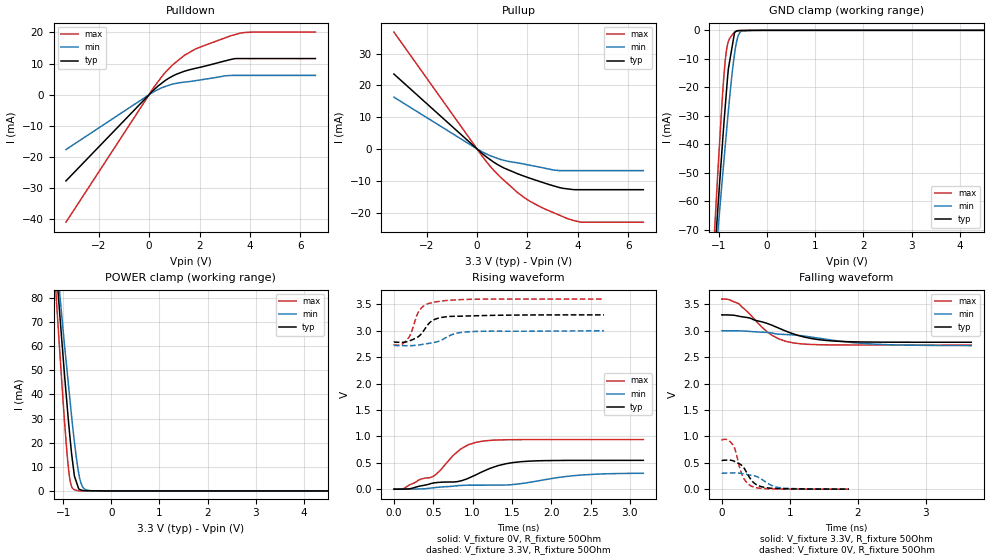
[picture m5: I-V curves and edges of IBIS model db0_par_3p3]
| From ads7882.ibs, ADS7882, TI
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|   db0_par_3p3 Model
[Model]   db0_par_3p3
Model_type   3-state
Polarity   Non-Inverting
Enable   Active-Low
Vmeas = 1.65
Vref = 1.65
Cref = 20pF
Rref = 50
|   typ   min   max
|   (nom PVT)   (Fast PVT)   (slow PVT)
|C_comp from frequency sweep method (F=1.5MHz)
|Average
C_comp   1.719e-12   1.545e-12   1.914e-12
|ON state : BUFFER OUTPUT TURNED HIGH
|C_comp   1.674e-12   1.503e-12   1.875e-12
|OFF state: BUFFER IN HIGH IMPEDANCE
|C_comp   1.764e-12   1.588e-12   1.953e-12
|C_comp from LC tank measurement(L=1nH)
|Resonant Frequency(Hz)   4.480e+09   4.600e+09   4.370e+09
|C_comp   1.263e-12   1.198e-12   1.328e-12
|ON state : BUFFER OUTPUT TURNED HIGH
|Resonant Frequency(Hz)   4.480e+09   4.600e+09   4.370e+09
|C_comp   1.263e-12   1.198e-12   1.328e-12
|OFF state: BUFFER IN HIGH IMPEDANCE
|Resonant Frequency   4.490e+09   4.600e+09   4.090e+09
|C_comp   1.258e-12   1.198e-12   1.516e-12
| Where nom  PVT is Nominal Process,  3.3V,  25C
|   Fast PVT is Strong Process,   3.6V,  -40C
|   Slow PVT is Weak Process,   3V,  85C
[Voltage Range]   3.3   3   3.6
|Ambient Temperature   25   85   -40
|Junction Temperature
[Temperature Range]   25   85   -40
[Pullup Reference]   3.3   3   3.6
[Pulldown Reference]   0   0   0
[Power Clamp Reference]   3.3   3   3.6
[GND Clamp Reference]   0   0   0
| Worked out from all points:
|   slope of the pulldown table from 0 to 0.495 V, typ, clamps not added: 135 ohm
|   slope of the pullup table from 0 to 0.495 V, typ, clamps not added: 154 ohm
|   GND clamp passes 1 mA (typ) near -0.68 V on its own axis
|   POWER clamp passes 1 mA (typ) near -0.68 V on its own axis
|   falling waveform, V_fixture 3.3V, R_fixture 50Ohm: 20-80 % time 703ps typ, 1.15ns min, 433ps max; typ from 3.3 V to 2.78 V
|   rising waveform, V_fixture 0V, R_fixture 50Ohm: 20-80 % time 826ps typ, 1.42ns min, 500ps max; typ from 0 V to 0.545 V
|   rising waveform, V_fixture 3.3V, R_fixture 50Ohm: 20-80 % time 185ps typ, 269ps min, 144ps max; typ from 2.78 V to 3.3 V
|   falling waveform, V_fixture 0V, R_fixture 50Ohm: 20-80 % time 178ps typ, 248ps min, 136ps max; typ from 0.546 V to 0 V
[Pulldown]
|   Voltage   I(typ)   I(min)   I(max)
-3.3V     -27.69mA   -17.63mA   -40.95mA
202.8mV   1.678mA    1.002mA    2.555mA
638.4mV   4.547mA    2.612mA    7.116mA
915.6mV   5.909mA    3.376mA    9.441mA
1.376V    7.461mA    4.003mA    12.49mA
1.916V    8.596mA    4.59mA     14.93mA
3.018V    10.85mA    6.05mA     18.25mA
3.432V    11.59mA    6.179mA    19.34mA
3.644V    11.59mA    6.179mA    19.82mA
4.127V    11.59mA    6.179mA    20.1mA
6.6V      11.59mA    6.179mA    20.1mA
[GND Clamp]
|   Voltage   I(typ)   I(min)   I(max)
-3.3V     -634.8mA   -537.3mA   -767.7mA
-1.136V   -90.43mA   -93.43mA   -83.87mA
-1.056V   -70.52mA   -77.1mA    -59.57mA
-1.01V    -59.08mA   -67.92mA   -45.7mA
-927.6mV  -39.68mA   -51.59mA   -22.91mA
-870mV    -26.75mA   -40.54mA   -10.58mA
-805.2mV  -13.53mA   -28.33mA   -3.894mA
-676.5mV  -750.2uA   -8.253mA   -729.3uA
-650.1mV  -330.5uA   -5.341mA   -460.8uA
-564mV    -97.6uA    -698.5uA   -56.58uA
-360mV    -55.08uA   -511.3nA   0A
6.6V      0A         0A         0A
[Pullup]
|   Voltage   I(typ)   I(min)   I(max)
-3.3V     23.55mA    16.29mA    36.76mA
202.8mV   -1.439mA   -906.1uA   -2.279mA
494.4mV   -3.213mA   -2.04mA    -5.205mA
915.6mV   -5.371mA   -3.274mA   -8.802mA
1.614V    -7.827mA   -4.388mA   -13.76mA
2.053V    -9.089mA   -5.062mA   -16.25mA
2.467V    -10.19mA   -5.705mA   -18.04mA
3.156V    -11.89mA   -6.741mA   -20.46mA
3.846V    -12.81mA   -6.823mA   -22.56mA
4.134V    -12.82mA   -6.823mA   -23.05mA
6.6V      -12.82mA   -6.823mA   -23.05mA
[POWER Clamp]
|   Voltage   I(typ)   I(min)   I(max)
-3.3V     660.3mA    569.4mA    775.2mA
-1.144V   92.02mA    97.34mA    80.17mA
-1.136V   90.18mA    95.79mA    77.92mA
-1.021V   60.73mA    71.04mA    42.87mA
-902.4mV  31.83mA    46.54mA    11.81mA
-852mV    20.98mA    36.39mA    3.781mA
-769.2mV  6.651mA    20.83mA    511.3uA
-696mV    2.004mA    9.587mA    107.3uA
-633mV    404.3uA    3.408mA    6.706uA
-567mV    133.2uA    945.8uA    0A
-429mV    94.19uA    74.67uA    0A
6.6V      0A         0A         0A
[Ramp]
R_load = 50
|   typ   min   max
dV/dt_r   0.327733/8.2648e-10   0.182281/1.43669e-09   0.563152/4.9974e-10
dV/dt_f   0.310442/7.02941e-10   0.168675/1.15224e-09   0.521793/4.32742e-10
[Falling Waveform]
V_fixture = 3.3V
V_fixture_min = 3V
V_fixture_max = 3.6V
R_fixture = 50Ohm
|   Time   V(typ)   V(min)   V(max)
0s        3.3V       3V         3.6V
103.9ps   3.299V     3V         3.592V
250.4ps   3.276V     2.998V     3.51V
674ps     3.136V     2.968V     2.973V
848.3ps   3.044V     2.935V     2.841V
1.048ns   2.943V     2.922V     2.772V
1.323ns   2.852V     2.879V     2.74V
1.723ns   2.8V       2.806V     2.732V
2.471ns   2.784V     2.735V     2.73V
3.671ns   2.783V     2.72V      2.73V
[Rising Waveform]
V_fixture = 0V
V_fixture_min = 0V
V_fixture_max = 0V
R_fixture = 50Ohm
|   Time   V(typ)   V(min)   V(max)
0s        2.808nV    7.638nV    2.658nV
118.6ps   401.9uV    -990.5nV   8.463mV
324.1ps   56.22mV    3.634mV    178.1mV
496.7ps   114.6mV    24.84mV    239.9mV
848.3ps   155.9mV    69.18mV    759.8mV
1.048ns   275.4mV    75.63mV    888.6mV
1.323ns   444.8mV    76.04mV    930.7mV
1.623ns   520.5mV    105.9mV    937.6mV
2.371ns   544.9mV    266mV      938mV
3.171ns   545.3mV    300.8mV    938.2mV
[Rising Waveform]
V_fixture = 3.3V
V_fixture_min = 3V
V_fixture_max = 3.6V
R_fixture = 50Ohm
|   Time   V(typ)   V(min)   V(max)
0s        2.783V     2.719V     2.73V
103.9ps   2.78V      2.718V     2.744V
180.5ps   2.798V     2.717V     2.855V
214.5ps   2.817V     2.717V     2.942V
287.1ps   2.867V     2.724V     3.274V
324.1ps   2.904V     2.732V     3.386V
466.4ps   3.169V     2.766V     3.525V
614.8ps   3.254V     2.831V     3.564V
919.5ps   3.278V     2.977V     3.592V
2.671ns   3.3V       2.999V     3.599V
[Falling Waveform]
V_fixture = 0V
V_fixture_min = 0V
V_fixture_max = 0V
R_fixture = 50Ohm
|   Time   V(typ)   V(min)   V(max)
0s        546.2mV    303.8mV    938.6mV
88.08ps   551mV      305.9mV    934.3mV
169.9ps   535.1mV    308.3mV    826.3mV
199.5ps   518mV      308.1mV    732.5mV
305.8ps   434.2mV    294.9mV    247.1mV
368.4ps   308.4mV    278.8mV    121.4mV
464.8ps   126.9mV    255.5mV    41.91mV
614.8ps   37.31mV    161.6mV    11.79mV
864.6ps   8.976mV    26.02mV    3.266mV
1.871ns   457.7uV    1.812mV    31.99uV
